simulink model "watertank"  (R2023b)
settings: Solver=ode3  StartTime=0.0  StopTime=1200  FixedStep=parSys.Ta  MaxStep=parSys.Ta  RelTol=1e-3  EnableMultiTasking=on
undefined symbols (not defined in the file or in its folder): parMHE, parSys, sigbuilder_block
libraries: simulink x3

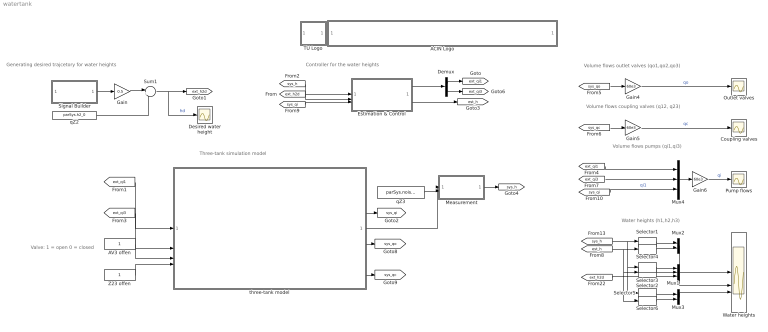
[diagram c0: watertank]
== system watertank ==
  note: Generating desired trajcetory for water heights
  note: Valve: 1 = open 0 = closed
  note: Volume flows outlet valves (qo1,qo2,qo3)
  note: Water heights (h1,h2,h3)
  note: Volume flows coupling valves (q12, q23)
  note: Volume flows pumps (qi1,qi3)
  note: Controller for the water heights
  note: Three-tank simulation model
  ACIN Logo : Subsystem
      mask init:
      | s = get_param(gcb,'UserData');
  AV3 offen : Constant
  Coupling valves : Scope
  Demux : Demux  Outputs=2
  Desired water height : Scope
  Estimation & Control : Subsystem
  Gain : Gain  Gain=0.5
  Gain4 : Gain  Gain=60e3
  Gain5 : Gain  Gain=60e3
  Gain6 : Gain  Gain=60e3
  Measurement : Subsystem
  Mux1 : Mux  Inputs=3
  Mux2 : Mux  Inputs=2
  Mux3 : Mux  Inputs=2
  Mux4 : Mux  Inputs=3
  Outlet valves : Scope
  Pump flows : Scope
  Selector1 : Selector  InputPortWidth=3  IndexOptions=Index vector (dialog)  Indices=1  OutputSizes=1
  Selector2 : Selector  InputPortWidth=3  IndexOptions=Index vector (dialog)  Indices=2  OutputSizes=1
  Selector3 : Selector  InputPortWidth=3  IndexOptions=Index vector (dialog)  Indices=2  OutputSizes=1
  Selector4 : Selector  InputPortWidth=3  IndexOptions=Index vector (dialog)  Indices=1  OutputSizes=1
  Selector5 : Selector  InputPortWidth=3  IndexOptions=Index vector (dialog)  Indices=3  OutputSizes=1
  Selector6 : Selector  InputPortWidth=3  IndexOptions=Index vector (dialog)  Indices=3  OutputSizes=1
  Signal Builder : Subsystem  Tag=STV Subsys  LoadFcn=sigbuilder_block('load');  StartFcn=sigbuilder_block('start');  StopFcn=sigbuilder_block('stop');  ClipboardFcn=sigbuilder_block('clipboard');  mask(Sigbuilder block){tuvar=[0:10]}
      mask help: Simulink:masks:SigbuilderBlock_MD
      mask init:
      | if ~strcmp(get_param(bdroot(gcbh),'SimulationStatus'),'stopped') tuvar = sigbuilder_block('maskInit'); end
  Sum1 : Sum  Inputs=|++
  TU Logo : Subsystem
      mask init:
      | s = get_param(gcb,'UserData');
  Water heights : Scope  NumInputPorts=3
  Z23 offen : Constant
  qZ2 : Constant  Value=parSys.h2_0
  qZ3 : Constant  Value=parSys.noise_on
  three-tank model : Subsystem
      mask init:
      | S = get_param(gcb,'UserData');
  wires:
  Sum1/1 -> Desired water height/1, [ext_h2d]  "hd"
  qZ2/1 -> Sum1/2
  Demux/1 -> [ext_qi1]
  Demux/2 -> [ext_qi3]
  three-tank model/4("[q12 q23]") -> [sys_qc]
  three-tank model/3("[qo1 qo2 qo3]") -> [sys_qo]
  Z23 offen/1 -> three-tank model/4(23)
  three-tank model/2("[qi1 qi3]") -> [sys_qi]
  three-tank model/1("[h1 h2 h3]") -> Measurement/1(h)
  Measurement/1(hmess) -> [sys_h]
  [ext_qi1] -> three-tank model/1(qi1)
  qZ3/1 -> Measurement/2(noise_on)
  AV3 offen/1 -> three-tank model/3(o3)
  [ext_qi3] -> three-tank model/2(qi3)
  Selector5/1 -> Mux3/1
  Mux4/1 -> Gain6/1
  Mux1/1 -> Water heights/2
  Selector1/1 -> Mux2/1
  Gain5/1 -> Coupling valves/1  "qc"
  Gain6/1 -> Pump flows/1  "qi"
  Selector3/1 -> Mux1/1
  [ext_h2d] -> Mux1/3
  [sys_qc] -> Gain5/1
  [sys_h] -> Selector5/1, Selector3/1, Selector1/1
  [sys_qo] -> Gain4/1
  Gain4/1 -> Outlet valves/1  "qo"
  [sys_qi] -> Mux4/3  "qi1"
  [ext_qi3] -> Mux4/2
  [ext_qi1] -> Mux4/1
  Gain/1 -> Sum1/1
  Signal Builder/1(Signal 2) -> Gain/1
  [sys_h] -> Estimation & Control/1(x)
  [ext_h2d] -> Estimation & Control/2(yref)
  Estimation & Control/1(u) -> Demux/1
  Estimation & Control/2(xEst) -> [est_h]
  Selector2/1 -> Mux1/2
  Selector4/1 -> Mux2/2
  Mux2/1 -> Water heights/1
  Mux3/1 -> Water heights/3
  Selector6/1 -> Mux3/2
  [est_h] -> Selector6/1, Selector2/1, Selector4/1
  [sys_qi] -> Estimation & Control/3(ureal)

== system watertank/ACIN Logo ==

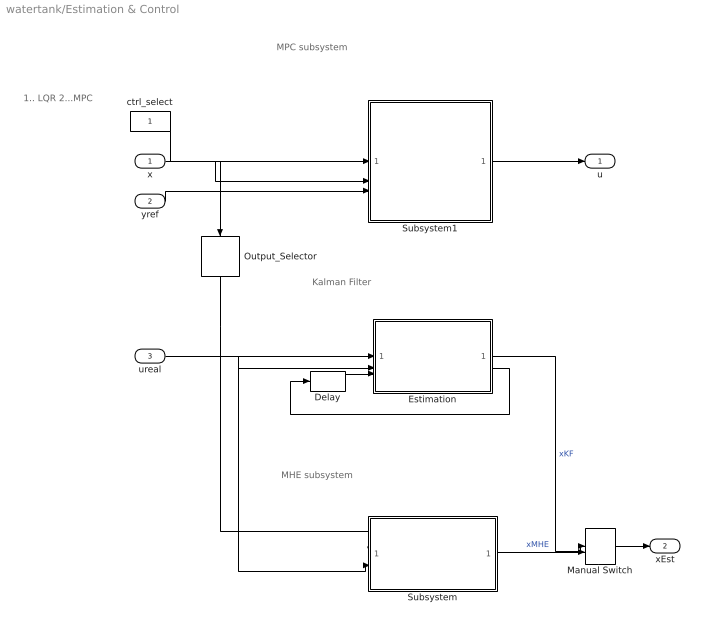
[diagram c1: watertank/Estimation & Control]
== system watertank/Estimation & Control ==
  note: Kalman Filter
  note: MHE subsystem
  note: MPC subsystem
  note: 1.. LQR 2...MPC
  x : Inport
  yref : Inport  Port=2
  ureal : Inport  Port=3
  Delay : Delay  DelayLength=1  InitialCondition=[0;0;0]
  Estimation : MATLAB Function  TreatAsAtomicUnit=on
  Manual Switch : ManualSwitch
  Output_Selector : Selector  InputPortWidth=3  IndexOptions=Index vector (dialog)  Indices=[1 3]  OutputSizes=1
  Subsystem : Subsystem
  Subsystem1 : Subsystem
  ctrl_select : Constant
  u : Outport
  xEst : Outport  Port=2
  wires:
  x/1 -> Output_Selector/1, Subsystem1/2(x)
  Delay/1 -> Estimation/3(dxm1)
  Estimation/2(dx) -> Delay/1
  ureal/1 -> Estimation/2(u), Subsystem/2(u)
  Output_Selector/1 -> Estimation/1(y), Subsystem/1(y)
  Subsystem/1(xEst) -> Manual Switch/2  "xMHE"
  Manual Switch/1 -> xEst/1
  Estimation/1(xEst) -> Manual Switch/1  "xKF"
  yref/1 -> Subsystem1/3(yref)
  Subsystem1/1(u) -> u/1
  ctrl_select/1 -> Subsystem1/1(ctrl switch)

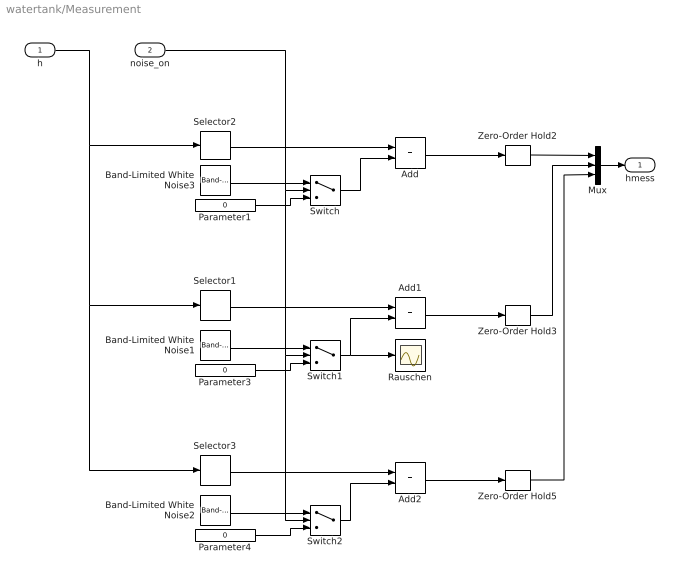
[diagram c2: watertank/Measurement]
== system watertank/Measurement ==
  h : Inport
  noise_on : Inport  Port=2
  Add : Sum
  Add1 : Sum
  Add2 : Sum
  Band-Limited White Noise1 : simulink/Sources/Band-Limited White Noise  Cov=parInit.meas.noisepow  Ts=parSys.Ts  seed=[981353]
  Band-Limited White Noise2 : simulink/Sources/Band-Limited White Noise  Cov=parInit.meas.noisepow  Ts=parSys.Ts  seed=[23343]
  Band-Limited White Noise3 : simulink/Sources/Band-Limited White Noise  Cov=parInit.meas.noisepow  Ts=parSys.Ts  seed=[23263]
  Mux : Mux  Inputs=3
  Parameter1 : Constant  Value=0  VectorParams1D=off
  Parameter3 : Constant  Value=0  VectorParams1D=off
  Parameter4 : Constant  Value=0  VectorParams1D=off
  Rauschen : Scope
  Selector1 : Selector  InputPortWidth=3  IndexOptions=Index vector (dialog)  Indices=[2]  OutputSizes=1
  Selector2 : Selector  InputPortWidth=3  IndexOptions=Index vector (dialog)  Indices=[1]  OutputSizes=1
  Selector3 : Selector  InputPortWidth=3  IndexOptions=Index vector (dialog)  Indices=[3]  OutputSizes=1
  Switch : Switch  Threshold=0.5
  Switch1 : Switch  Threshold=0.5
  Switch2 : Switch  Threshold=0.5
  Zero-Order Hold2 : ZeroOrderHold  SampleTime=parSys.Ts
  Zero-Order Hold3 : ZeroOrderHold  SampleTime=parSys.Ts
  Zero-Order Hold5 : ZeroOrderHold  SampleTime=parSys.Ts
  hmess : Outport  VectorParamsAs1DForOutWhenUnconnected=off
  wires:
  Band-Limited White Noise3/1 -> Switch/1
  Switch/1 -> Add/2
  noise_on/1 -> Switch/2, Switch1/2, Switch2/2
  Selector2/1 -> Add/1
  Parameter1/1 -> Switch/3
  Band-Limited White Noise1/1 -> Switch1/1
  Switch1/1 -> Rauschen/1, Add1/2
  Selector1/1 -> Add1/1
  Parameter3/1 -> Switch1/3
  Band-Limited White Noise2/1 -> Switch2/1
  Switch2/1 -> Add2/2
  Parameter4/1 -> Switch2/3
  Add/1 -> Zero-Order Hold2/1
  Add1/1 -> Zero-Order Hold3/1
  Add2/1 -> Zero-Order Hold5/1
  Selector3/1 -> Add2/1
  h/1 -> Selector1/1, Selector3/1, Selector2/1
  Mux/1 -> hmess/1
  Zero-Order Hold2/1 -> Mux/1
  Zero-Order Hold3/1 -> Mux/2
  Zero-Order Hold5/1 -> Mux/3

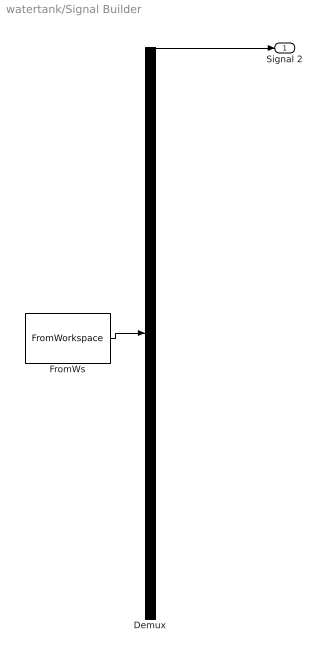
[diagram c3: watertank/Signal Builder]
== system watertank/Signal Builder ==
  Demux : Demux  Tag=STV Demux  Outputs=1
  FromWs : FromWorkspace  Tag=STV FromWs  VariableName=tuvar
  Signal 2 : Outport  Tag=STV Outport  VectorParamsAs1DForOutWhenUnconnected=off
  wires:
  FromWs/1 -> Demux/1
  Demux/1 -> Signal 2/1

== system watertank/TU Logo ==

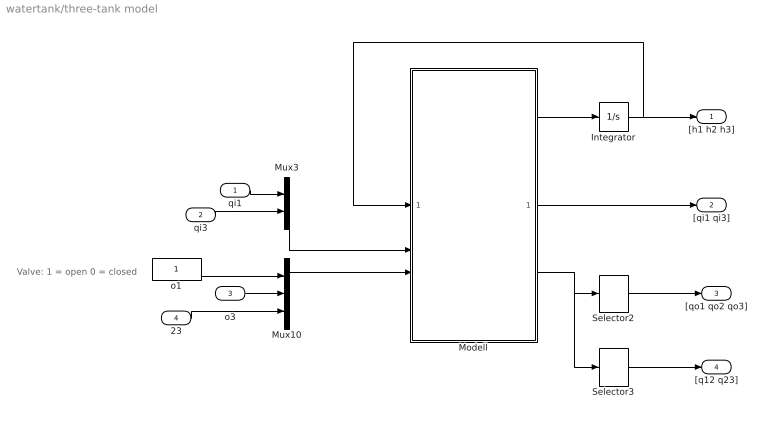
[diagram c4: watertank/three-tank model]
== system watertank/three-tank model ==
  note: Valve: 1 = open 0 = closed
  qi1 : Inport
  qi3 : Inport  Port=2
  o3 : Inport  Port=3
  23 : Inport  Port=4
  Integrator : Integrator  InitialCondition=[parSys.h1_0; parSys.h2_0; parSys.h3_0]
  Modell : MATLAB Function  TreatAsAtomicUnit=on
  Mux10 : Mux  Inputs=3
  Mux3 : Mux  Inputs=2
  Selector2 : Selector  InputPortWidth=5  IndexOptions=Index vector (dialog)  Indices=[1 2 3]  OutputSizes=1
  Selector3 : Selector  InputPortWidth=5  IndexOptions=Index vector (dialog)  Indices=[4 5]  OutputSizes=1
  o1 : Constant
  "[h1 h2 h3]" : Outport  VectorParamsAs1DForOutWhenUnconnected=off
  "[qi1 qi3]" : Outport  Port=2  VectorParamsAs1DForOutWhenUnconnected=off
  "[qo1 qo2 qo3]" : Outport  Port=3  VectorParamsAs1DForOutWhenUnconnected=off
  "[q12 q23]" : Outport  Port=4  VectorParamsAs1DForOutWhenUnconnected=off
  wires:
  o1/1 -> Mux10/1
  qi1/1 -> Mux3/1
  qi3/1 -> Mux3/2
  Selector2/1 -> "[qo1 qo2 qo3]"/1
  Selector3/1 -> "[q12 q23]"/1
  23/1 -> Mux10/3
  o3/1 -> Mux10/2
  Mux10/1 -> Modell/3(is_open)
  Modell/1(dx) -> Integrator/1
  Integrator/1 -> Modell/1(x), "[h1 h2 h3]"/1
  Mux3/1 -> Modell/2(qi)
  Modell/3(q_valve) -> Selector3/1, Selector2/1
  Modell/2(q_pump) -> "[qi1 qi3]"/1

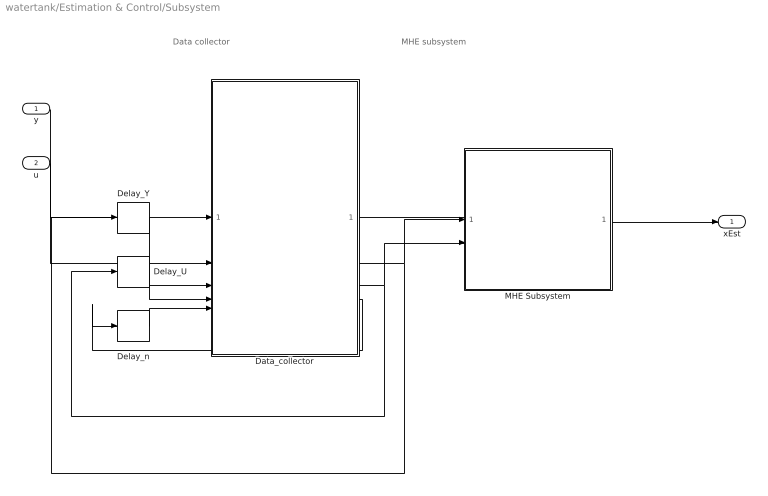
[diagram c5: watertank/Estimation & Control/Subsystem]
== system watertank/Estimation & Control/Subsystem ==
  note: Data collector
  note: MHE subsystem
  y : Inport
  u : Inport  Port=2
  Data_collector : MATLAB Function  TreatAsAtomicUnit=on
  Delay_U : Delay  DelayLength=1  InitialCondition=zeros(parMHE.N*parMHE.n_u,1)
  Delay_Y : Delay  DelayLength=1  InitialCondition=zeros(parMHE.N*parMHE.n_y,1)
  Delay_n : Delay  DelayLength=1
  MHE Subsystem : Subsystem  TreatAsAtomicUnit=on
  xEst : Outport
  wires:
  Data_collector/4(cnt) -> Delay_n/1
  Delay_n/1 -> Data_collector/5(cnt_m1)
  Delay_U/1 -> Data_collector/4(U_collected_m1)
  u/1 -> Data_collector/2(u)
  MHE Subsystem/1(x_est) -> xEst/1
  Data_collector/3(U_collected) -> Delay_U/1, MHE Subsystem/2(u_collected)
  Delay_Y/1 -> Data_collector/3(Y_collected_m1)
  Data_collector/1(enable) -> MHE Subsystem/Enable
  y/1 -> Data_collector/1(y)
  Data_collector/2(Y_collected) -> Delay_Y/1, MHE Subsystem/1(y_collected)

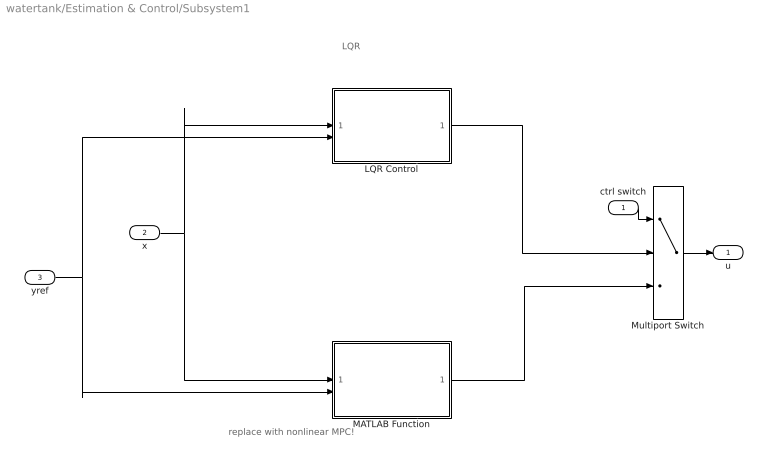
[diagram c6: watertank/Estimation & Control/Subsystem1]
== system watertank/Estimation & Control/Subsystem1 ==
  note: LQR
  note: replace with nonlinear MPC!
  ctrl switch : Inport
  x : Inport  Port=2
  yref : Inport  Port=3
  LQR Control : MATLAB Function  TreatAsAtomicUnit=on
  MATLAB Function : MATLAB Function  TreatAsAtomicUnit=on
  Multiport Switch : MultiPortSwitch  Inputs=2
  u : Outport
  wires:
  yref/1 -> MATLAB Function/2(y_ref), LQR Control/2(yref)
  LQR Control/1(u) -> Multiport Switch/2
  x/1 -> LQR Control/1(x), MATLAB Function/1(x)
  Multiport Switch/1 -> u/1
  ctrl switch/1 -> Multiport Switch/1
  MATLAB Function/1(u) -> Multiport Switch/3

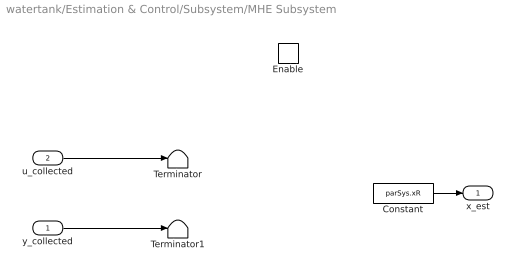
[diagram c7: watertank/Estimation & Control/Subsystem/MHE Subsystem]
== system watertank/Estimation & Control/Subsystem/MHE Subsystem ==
  y_collected : Inport
  u_collected : Inport  Port=2
  Enable : EnablePort
  Constant : Constant  Value=parSys.xR
  Terminator : Terminator
  Terminator1 : Terminator
  x_est : Outport  InitialOutput=[parSys.xR]
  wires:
  y_collected/1 -> Terminator1/1
  u_collected/1 -> Terminator/1
  Constant/1 -> x_est/1

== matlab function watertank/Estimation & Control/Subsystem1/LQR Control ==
function u    = fcn(x, yref, parSys)
% LQR based on the linearized discrete-time dynamics

% Calculate total control input
u = parSys.uR + parSys.K * x + parSys.f * yref;

end

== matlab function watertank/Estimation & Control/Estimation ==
function [xEst,dx] = fcn(y, u, dxm1, parSys)
% Kalman filter based on the linearized discrete-time dynamics

% Write output
xEst = dxm1 + parSys.xR;

% Update state estimation
dx = parSys.Ad * dxm1 + parSys.Bd * (u - parSys.uR) + parSys.Kkal * (y - parSys.Cd * xEst);

end

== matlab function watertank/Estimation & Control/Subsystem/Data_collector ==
function [enable, Y_collected, U_collected, cnt] = fcn(y, u, Y_collected_m1, U_collected_m1, cnt_m1, parMHE)
% Data collector for MHE estimation

% Increase counter of recieved data points
cnt = cnt_m1 + 1;

% Assemble vector of recieved output measurements
Y_collected = [Y_collected_m1(parMHE.n_y+1:end,1); y(:)];

% Assemble vector of recieven input values
U_collected = [U_collected_m1(parMHE.n_u+1:end,1); u(:)];

% Set enable flag for MHE if sufficient data is collected
if cnt >= parMHE.N
    enable = 1;
else
    enable = 0;
end

end

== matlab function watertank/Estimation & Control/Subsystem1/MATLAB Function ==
function u = MPC_template(x,y_ref)

u = y_ref;

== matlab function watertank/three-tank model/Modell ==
function [dx, q_pump, q_valve] = fcn(x, qi, is_open, parSys)
%#codegen

[dx, q_pump, q_valve] = watertank_mfun(x, qi, is_open, parSys);

% Function end
end
